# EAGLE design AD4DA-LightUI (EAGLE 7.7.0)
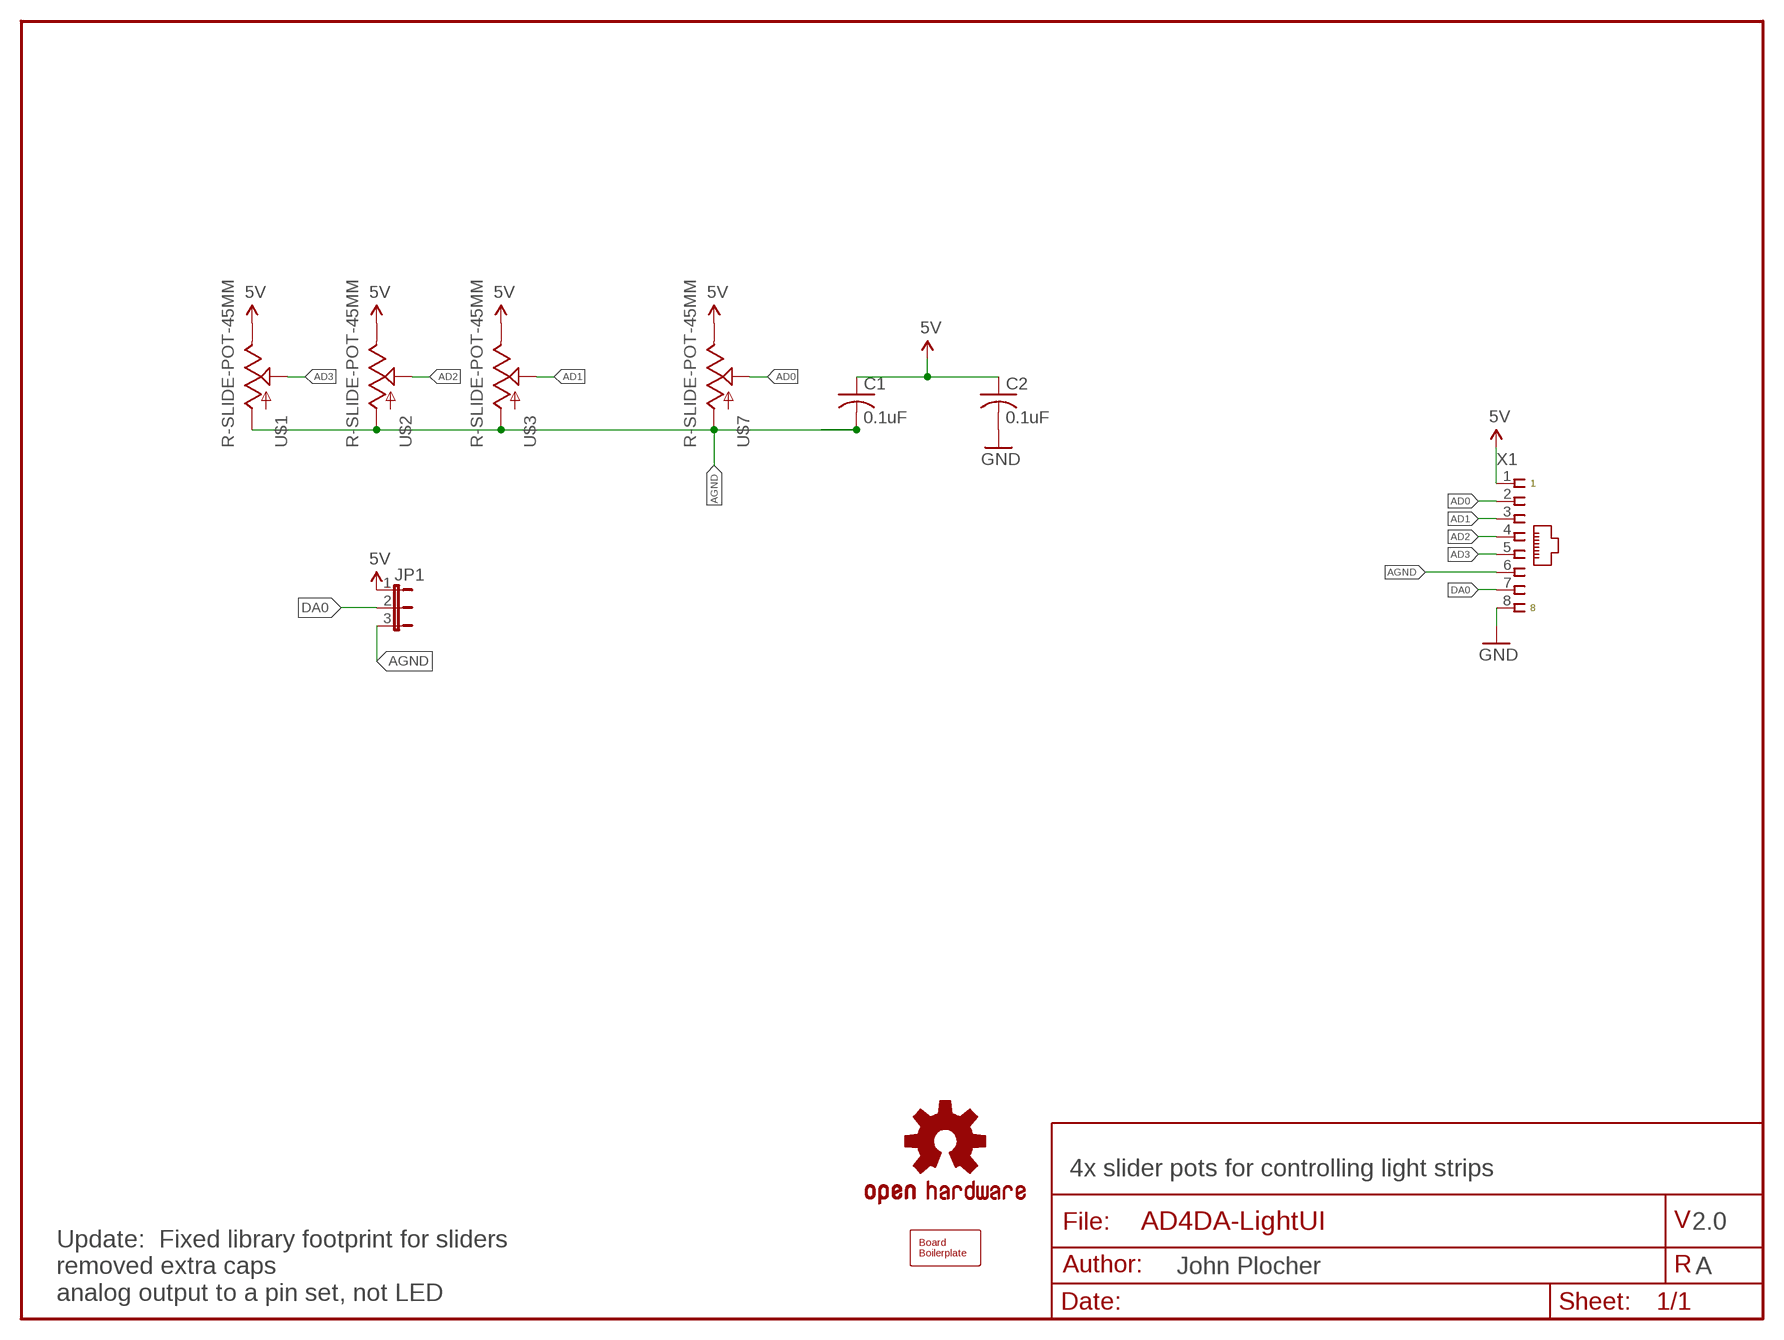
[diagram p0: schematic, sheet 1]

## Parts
C1  0.1uF  CAPPTH1  [C050-024X044]
C2  0.1uF  CAPPTH1  [C050-024X044]
JP1  JUMPER-3PTH-LOCK  [1X03]
LOGO1  DOC-OSHW-LOGO-L  [OSHW-LOGO-L]
U$1  R-SLIDE-POT-45MM  [SLIDER-45MM]
U$2  R-SLIDE-POT-45MM  [SLIDER-45MM]
U$3  R-SLIDE-POT-45MM  [SLIDER-45MM]
U$7  R-SLIDE-POT-45MM  [SLIDER-45MM]
U$9  BOARD80X100  [BOARD-DINRAIL-3.17INX10CM]
X1  CONNECTOR-RJ45-FRONT  [RJ45-NO-SHIELD]

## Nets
5V: C1.1 C2.1 JP1.1 U$1.E U$2.E U$3.E U$7.E X1.1
AD0: U$7.S X1.2
AD1: U$3.S X1.3
AD2: U$2.S X1.4
AD3: U$1.S X1.5
AGND: C1.2 JP1.3 U$1.A U$2.A U$3.A U$7.A X1.6
DA0: JP1.2 X1.7
GND: C2.2 X1.8

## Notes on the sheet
- 4x slider pots for controlling light strips
- 2.0
- A
- Update:  Fixed library footprint for sliders
  removed extra caps
  analog output to a pin set, not LED

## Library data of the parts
C1 C2 = SPCoast:CAP*
JP1 = SPCoast:JUMPER-3
LOGO1 = SPCoast:DOC-OSHW-LOGO-: Open Source Hardware Logo
U$1-U$3 U$7 = SPCoast:R-SLIDE-POT: Slide-type potentiometer- COM-9119
U$9 = SPCoast:BOARD
X1 = SPCoast:CONNECTOR-RJ45: Tyco CORCOM Modular RJ Jacks No Shield; AMP: 520151-4; OPL: none

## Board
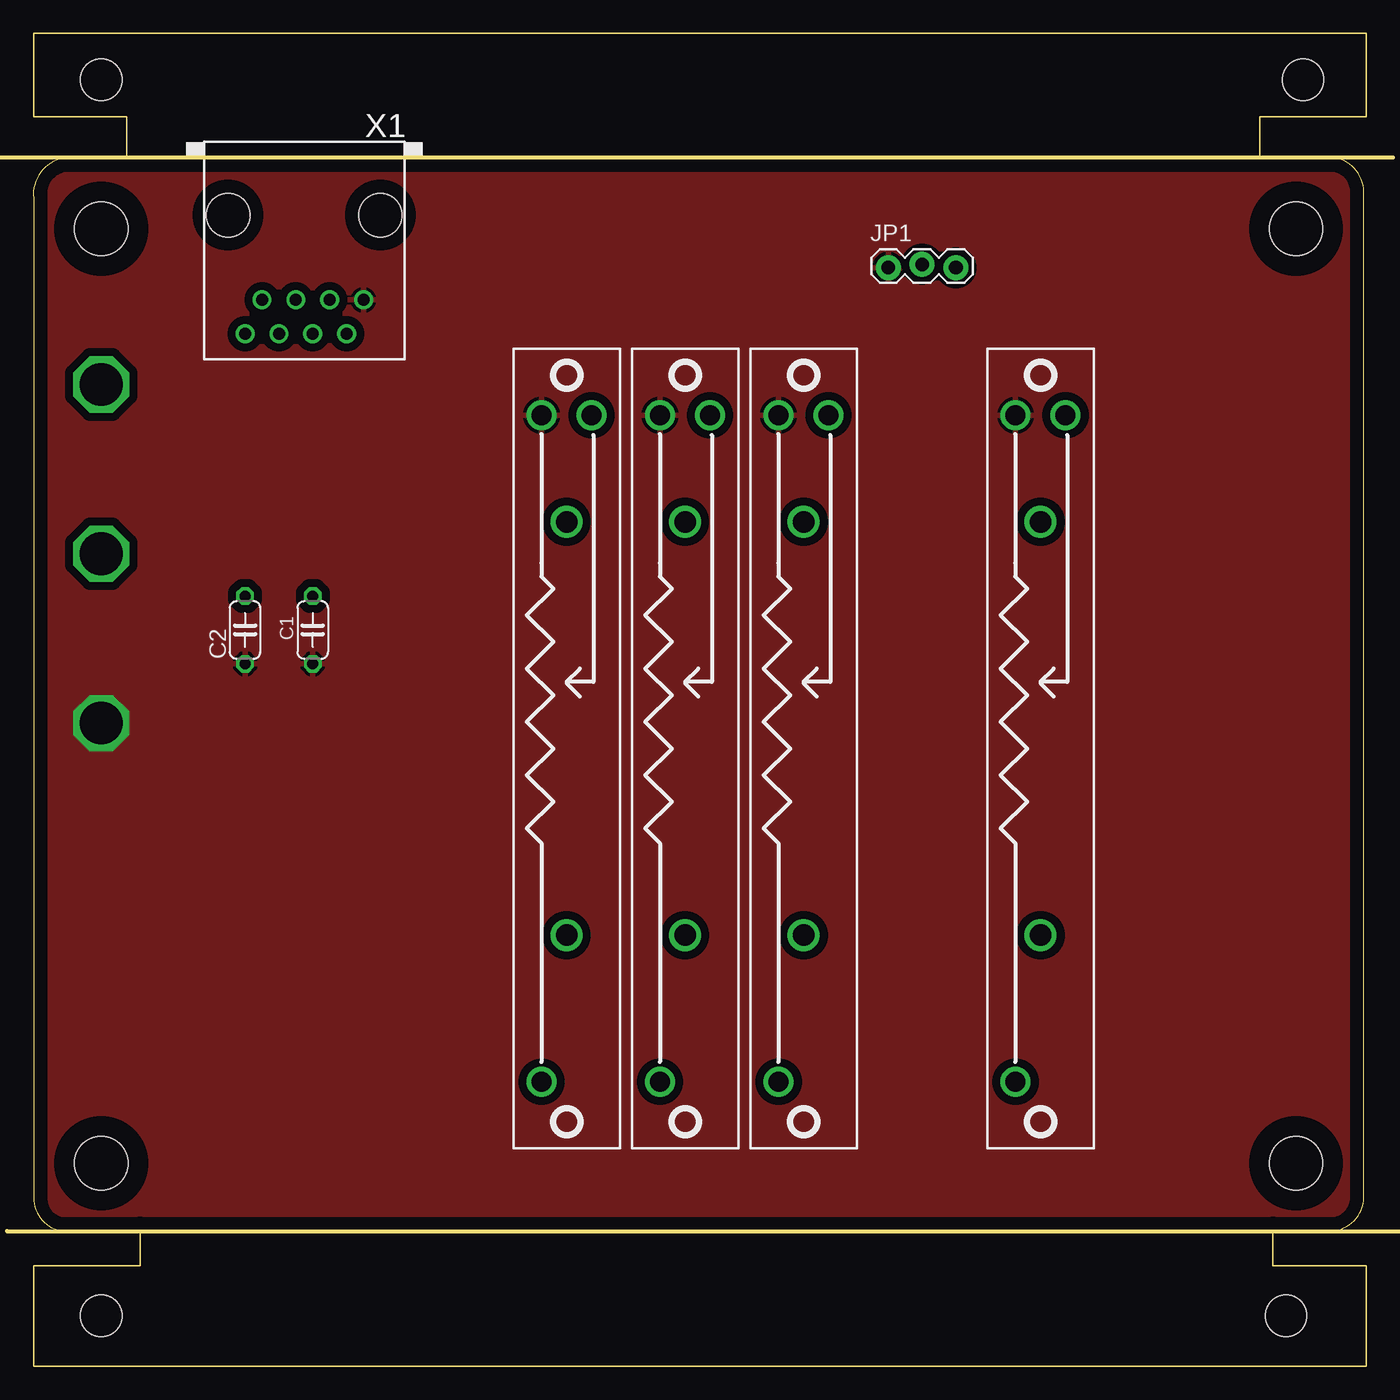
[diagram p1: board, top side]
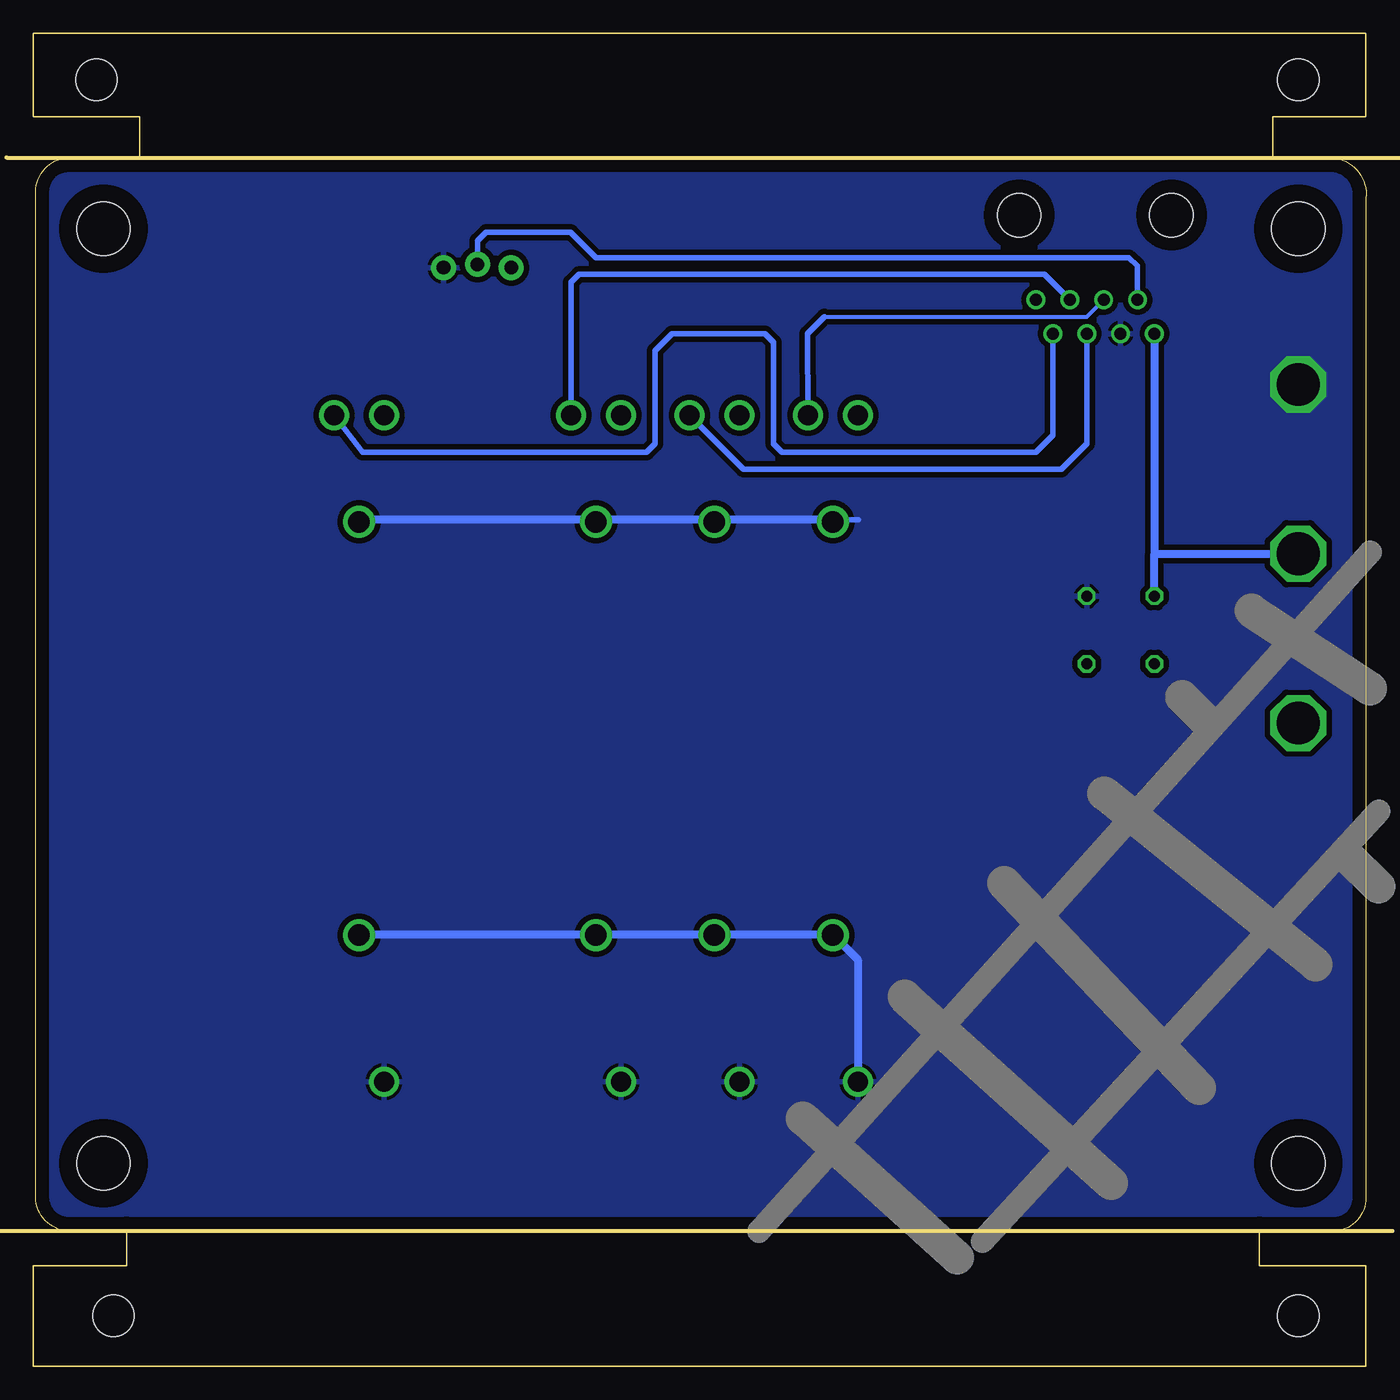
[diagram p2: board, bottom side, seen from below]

Size 100.01 x 100 mm. Coordinates in mm from the lower left corner, seen from the top.
Copper layers (1*16): Top 0.035mm / dielectric 1.5mm / Bottom 0.035mm
Design rules "default": minimum track width 10mil, minimum drill 0.6mm, track to track 8mil, track to pad 8mil, pad to pad 8mil, via to via 8mil, smd to smd 8mil, copper to edge 40mil, drill to drill 8mil, minimum pad ring 10mil, minimum via ring 8mil, stop-mask expansion 4mil, vias tented up to drill 0mil, thermal gap 10mil

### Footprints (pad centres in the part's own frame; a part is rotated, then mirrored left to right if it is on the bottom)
C050-024X044 = drill 0.813 octagon: 1 -2.54,0; 2 2.54,0
1X03 = drill 1.016 pad 1.88: 1 0,-0.127; 2 2.54,0.127; 3 5.08,-0.127
SLIDER-45MM = drill 1.5: A 25,-1.875; E -25,-1.875; S -25,1.875 | drill 1.6: G@0 -17,0; G@1 14,0
BOARD-DINRAIL-3.17INX10CM = hole 4: 94.742,15.24; 5.08,85.344; 94.742,85.344; 5.08,15.24 | hole 3.1: 5.08,96.52; 95.25,96.52; 5.08,3.81; 93.98,3.81
RJ45-NO-SHIELD = drill 0.9 pad 1.4: 1 -4.445,6.35; 2 -3.175,8.89; 3 -1.905,6.35; 4 -0.635,8.89; 5 0.635,6.35; 6 1.905,8.89; 7 3.175,6.35; 8 4.445,8.89 | hole 3.251: -5.715,0; 5.715,0

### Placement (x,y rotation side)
C1  20.97,55.24 90 top
C2  15.89,55.24 90 top
JP1  64.15,82.55 0 top
LOGO1  5.09,85.09 0 top
U$1  40.02,46.35 270 top
U$2  48.91,46.35 270 top
U$3  57.8,46.35 270 top
U$7  75.58,46.35 270 top
U$9  0.01,0 0 top
X1  20.33,86.36 180 top

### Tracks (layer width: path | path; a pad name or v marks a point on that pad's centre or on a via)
5V  (via drill 3.2)
  other vias: 5.09,48.26
  pour Top (isolate 0.61): 0.01,89.41 100.09,89.41 100.09,11.43 0.01,11.43
AD0
  Bottom 0.406: U$7.S 75.31,68.58 53.99,68.58 53.35,69.22 53.35,76.2 52.08,77.47 45.1,77.47 44.46,76.83 44.46,69.22 43.83,68.58 24.78,68.58 23.51,69.85 X1.2
AD1
  Bottom 0.406: X1.3 24.14,81.92 59.07,81.92 59.67,81.31 U$3.S
AD2
  Bottom 0.406: U$2.S 46.74,67.31 22.87,67.31 20.97,69.22 X1.4
AD3
  Bottom 0.305: 40.65,78.74 20.97,78.74 X1.5
  Bottom 0.406: U$1.S 41.92,77.47 40.65,78.74
AGND  (via drill 3.2)
  Bottom 0.406: 40.02,63.5 38.11,63.5
  Bottom 0.61: 75.58,32.38 40.02,32.38 38.14,30.51 U$1.A | 40.02,63.5 75.58,63.5
  other vias: 5.09,73.66
  pour Bottom (isolate 0.406): 0.01,89.41 100.09,89.41 100.09,11.43 0.01,11.43
DA0
  Bottom 0.406: X1.7 17.16,82.55 17.79,83.19 57.8,83.19 59.7,85.09 66.05,85.09 66.69,84.45 JP1.2
GND  (via drill 3.2)
  Bottom 0.61: X1.8 15.89,60.96 | 15.89,60.96 v5.09,60.96 | C2.2 15.89,60.96

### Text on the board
tDocu: v2.0 | D/A out | R G B | White | AD2 | OSHW / John Plocher | +5 | AD3 | AD1 | DA0 | Agnd | AD0 | DA0 | AD3 | AD2 | AD1 | AD0 | +5 | +5 | Dgnd | Agnd | Dgnd | LightUI | Agnd | 2014-11 B
bDocu: Made in the PCR, Coast Division, NMRA | LightUI | Solder Side | Go Bears! | Model Railroading is fun! | www . SPCoast . com
Changes: Slide pot had incorrect pin spacing

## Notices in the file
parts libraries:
SparkFun-Aesthetics: Licensing: CC v3.0 Share-Alike You are welcome to use this library for commercial purposes.
SPCoast: http://freedomdefined.org/OSHW Creative Commons - Attribution - ShareAlike 3.0
